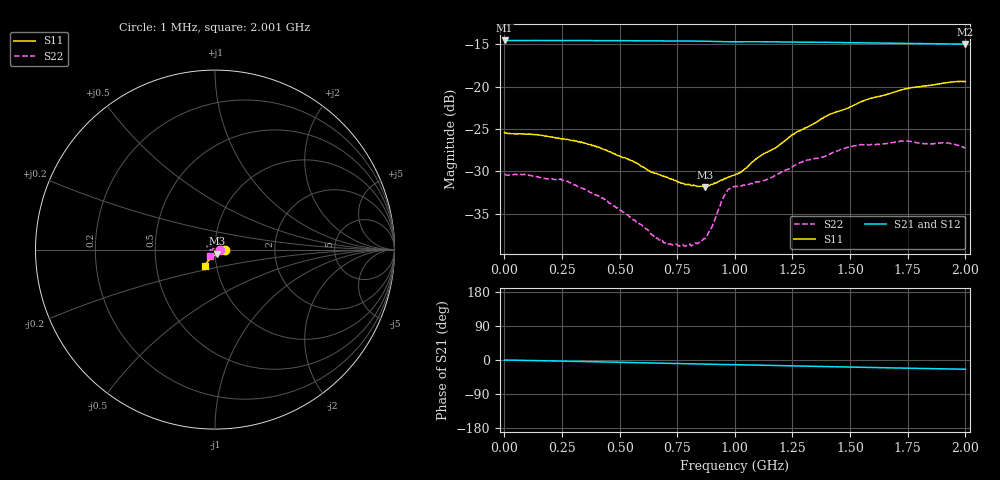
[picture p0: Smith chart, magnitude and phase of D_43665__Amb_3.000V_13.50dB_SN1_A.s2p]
! device id: 43665_
! dir: \\malibu\benchdata\1_engineers\tn_data\43665_75ohm\new\sparar\43665_\amb\3p000v\13p50db
! Serial: 1
! Insertion: A
! Temp: Amb
! VDD: 3.000V
! Attenuation Step: 13.50dB
! IDD: 1.442628e+00mA
! FILE NAME
! DATE 03-27-2009 08:36:40
! CORRECTED  DATA
#  Hz  S  RI  R  75
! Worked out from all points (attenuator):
!   401 points, 1 MHz to 2.001 GHz, reference 75 ohm
!   highest |S21| = -14.57 dB at 1 MHz (marker M1); lowest = -15.0 dB at 2.001 GHz (marker M2)
!   lowest |S11| = -31.8 dB at 871 MHz (marker M3), VSWR 1.05, Z = 76.6 - j3.52 ohm
!   |S11| at or under -10 dB: start of sweep to end of sweep
!   |S22| runs from -38.8 to -26.4 dB; largest |S21 - S12| = 0.0006
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1000000  0.0537 -0.00059  0.1869 -0.000419  0.187 -0.000268  0.0304 -0.000242
2.36e8  0.0496 -0.00304  0.1865 -0.00908  0.1865 -0.00908  0.0265 0.0104
3.36e8  0.047 -0.00492  0.1861 -0.013  0.1862 -0.013  0.0212 0.0137
4.26e8  0.0423 -0.00659  0.1857 -0.0165  0.1858 -0.0165  0.0166 0.0147
6.01e8  0.0316 -0.0116  0.1844 -0.0235  0.1844 -0.0235  0.0042 0.0144
6.71e8  0.0267 -0.0145  0.1839 -0.0263  0.184 -0.0263  0.000461 0.0125
7.21e8  0.0233 -0.0166  0.1836 -0.0284  0.1836 -0.0283  -0.00238 0.0116
7.91e8  0.0182 -0.0193  0.1828 -0.0314  0.1828 -0.0313  -0.00772 0.00861
8.31e8  0.0149 -0.0214  0.1823 -0.0331  0.1823 -0.033  -0.0105 0.0058
8.71e8  0.0113 -0.023  0.1816 -0.0349  0.1817 -0.0348  -0.0125 0.00225
9.01e8  0.00842 -0.0252  0.1809 -0.0362  0.181 -0.036  -0.0149 -0.000156
9.61e8  0.00343 -0.0285  0.1796 -0.0378  0.1797 -0.0376  -0.0235 -0.00162
1.001e9  0.000275 -0.0302  0.1795 -0.0388  0.1796 -0.0387  -0.0258 -0.000733
1.141e9  -0.0121 -0.0392  0.178 -0.0446  0.1782 -0.0444  -0.0273 -0.00788
1.261e9  -0.0229 -0.0479  0.176 -0.0493  0.1763 -0.0492  -0.0303 -0.0163
1.336e9  -0.0282 -0.0527  0.1749 -0.0519  0.1753 -0.0517  -0.0315 -0.0201
1.411e9  -0.0342 -0.0594  0.1736 -0.055  0.174 -0.055  -0.0307 -0.0256
1.511e9  -0.0411 -0.0651  0.1716 -0.0583  0.1719 -0.0583  -0.0332 -0.0296
1.671e9  -0.0495 -0.0761  0.1685 -0.0637  0.1686 -0.0639  -0.0317 -0.0339
1.736e9  -0.0525 -0.081  0.1671 -0.0658  0.1674 -0.066  -0.0309 -0.0365
1.916e9  -0.0573 -0.0883  0.1636 -0.071  0.1637 -0.0711  -0.0287 -0.0366
2.001e9  -0.0573 -0.0904  0.1619 -0.0733  0.1616 -0.0738  -0.0258 -0.035
